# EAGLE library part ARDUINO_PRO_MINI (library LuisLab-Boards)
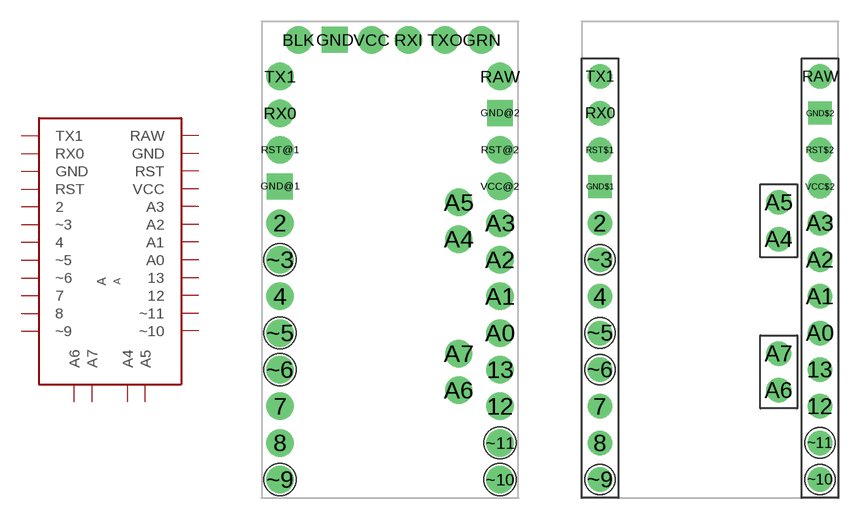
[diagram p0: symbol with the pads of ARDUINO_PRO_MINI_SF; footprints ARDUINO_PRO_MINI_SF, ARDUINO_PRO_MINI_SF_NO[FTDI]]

Designator prefix A

## ARDUINO_PRO_MINI_FTDI  [ARDUINO_PRO_MINI_SF]
2  2
4  4
7  7
8  8
12  12
13  13
A0  A0
A1  A1
A2  A2
A3  A3
A4  A4
A5  A5
A6  A6
A7  A7
GND@1  GND
GND@2  GND
RAW  RAW
RST@1  RST
RST@2  RST
RX0  RX0
TX1  TX1
VCC@2  VCC
~3  ~3
~5  ~5
~6  ~6
~9  ~9
~10  ~10
~11  ~11

## ARDUINO_PRO_MINI_NO-FTDI  [ARDUINO_PRO_MINI_SF_NO[FTDI]]
2  2
4  4
7  7
8  8
12  12
13  13
A0  A0
A1  A1
A2  A2
A3  A3
A4  A4
A5  A5
A6  A6
A7  A7
GND$1  GND
GND$2  GND
RAW  RAW
RST$1  RST
RST$2  RST
RX0  RX0
TX1  TX1
VCC$2  VCC
~3  ~3
~5  ~5
~6  ~6
~9  ~9
~10  ~10
~11  ~11

## Footprint ARDUINO_PRO_MINI_SF (pad centres in mm)
Arduino Pro Mini by SparkFun with FTDI Serial TTL pads. Available in 5V and 3.3V versions.
drill 1 pad 1.9: 2 -7.62,2.54; 4 -7.62,-2.54; 7 -7.62,-10.16; 8 -7.62,-12.7; 12 7.62,-10.16; 13 7.62,-7.62; A0 7.62,-5.08; A1 7.62,-2.54; A2 7.62,0; A3 7.62,2.54; A4 4.763,1.429; A5 4.763,3.969; A6 4.763,-9.049; A7 4.763,-6.509; BLK -6.35,15.24; GRN 6.35,15.24; RAW 7.62,12.7; RST@1 -7.62,7.62; RST@2 7.62,7.62; RX0 -7.62,10.16; RXI 1.27,15.24; TX1 -7.62,12.7; TXO 3.81,15.24; VCC -1.27,15.24; VCC@2 7.62,5.08; ~3 -7.62,0; ~5 -7.62,-5.08; ~6 -7.62,-7.62; ~9 -7.62,-15.24; ~10 7.62,-15.24; ~11 7.62,-12.7
drill 1 pad 1.8 square: GND -3.81,15.24; GND@1 -7.62,5.08; GND@2 7.62,10.16

## Footprint ARDUINO_PRO_MINI_SF_NO[FTDI] (pad centres in mm)
Arduino Pro Mini by SparkFun without FTDI Serial TTL pads. Available in 5V and 3.3V versions.
drill 1.016 pad 1.7: 2 -7.62,2.54; 4 -7.62,-2.54; 7 -7.62,-10.16; 8 -7.62,-12.7; 12 7.62,-10.16; 13 7.62,-7.62; A0 7.62,-5.08; A1 7.62,-2.54; A2 7.62,0; A3 7.62,2.54; A4 4.763,1.429; A5 4.763,3.969; A6 4.763,-9.049; A7 4.763,-6.509; RAW 7.62,12.7; RST$1 -7.62,7.62; RST$2 7.62,7.62; RX0 -7.62,10.16; TX1 -7.62,12.7; VCC$2 7.62,5.08; ~3 -7.62,0; ~5 -7.62,-5.08; ~6 -7.62,-7.62; ~9 -7.62,-15.24; ~10 7.62,-15.24; ~11 7.62,-12.7
drill 1.016 pad 1.6 square: GND$1 -7.62,5.08; GND$2 7.62,10.16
